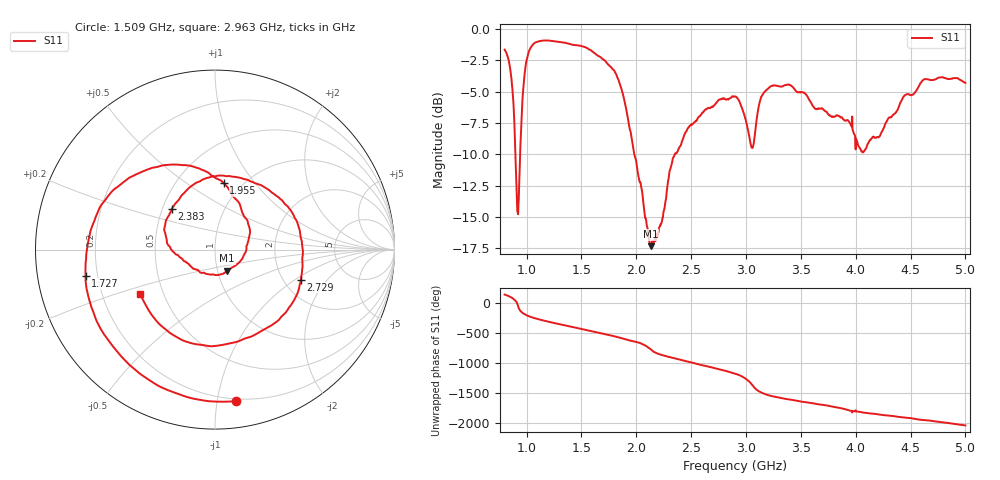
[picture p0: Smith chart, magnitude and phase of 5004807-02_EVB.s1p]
#  HZ  S  RI  R  50.00
! Rohde & Schwarz ZVA/B
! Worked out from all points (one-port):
!   1601 points, 800 MHz to 5 GHz, reference 50 ohm
!   lowest |S11| = -17.3 dB at 2.134 GHz (marker M1), VSWR 1.31, Z = 55.5 - j13.3 ohm
!   |S11| at or under -10 dB: 898.3 MHz to 940.9 MHz (42.58 MHz wide, 4.63 % of centre); 1.982 GHz to 2.351 GHz (369.7 MHz wide, 17.1 % of centre)
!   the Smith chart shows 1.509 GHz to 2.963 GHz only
!   S11 on the Smith chart (normalised r, x): 1.509 GHz: 0.18, -1.13; 1.727 GHz: 0.15, -0.10; 1.955 GHz: 0.83, +0.71; 2.383 GHz: 0.56, +0.28; 2.729 GHz: 2.47, -1.12; 2.963 GHz: 0.37, -0.24
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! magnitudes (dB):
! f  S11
! 800 MHz  -1.7
! 863 MHz  -4.0
! 907.6 MHz  -12.7
! 920.8 MHz  -14.7
! 933.9 MHz  -12.3
! 973.2 MHz  -4.4
! 1.018 GHz  -1.9
! 1.325 GHz  -1.1
! 1.509 GHz  -1.4
! 1.727 GHz  -2.7
! 1.85 GHz  -4.4
! 1.955 GHz  -8.6
! 2.134 GHz  -17.3
! 2.215 GHz  -15.8
! 2.317 GHz  -11.0
! 2.375 GHz  -9.8
! 2.383 GHz  -9.6
! 2.729 GHz  -5.9
! 2.9 GHz  -5.4
! 2.963 GHz  -6.3
! 3.058 GHz  -9.5
! 3.16 GHz  -5.1
! 3.425 GHz  -4.6
! 3.95 GHz  -7.6
! 4.071 GHz  -9.8
! 4.475 GHz  -5.2
! 4.635 GHz  -4.0
! 5 GHz  -4.3
